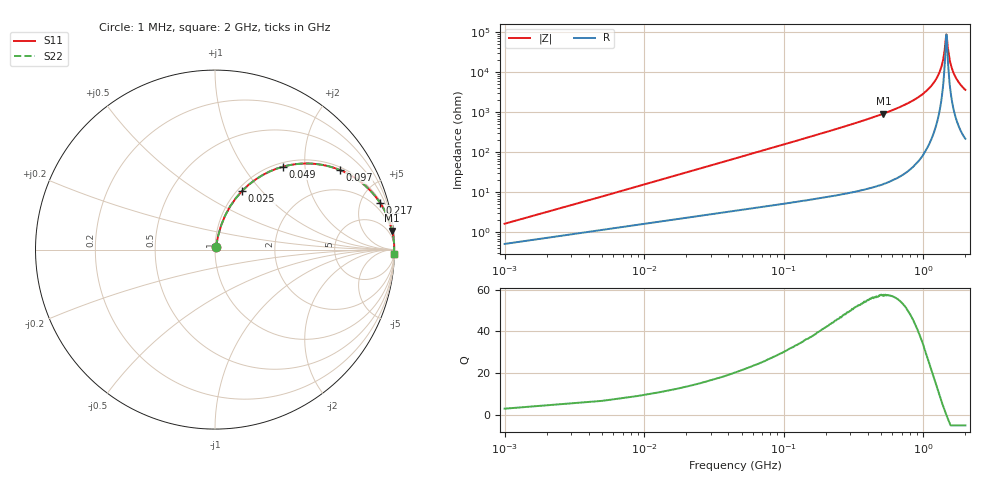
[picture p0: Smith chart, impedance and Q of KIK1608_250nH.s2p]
!version-2
!date-01.2022
!Series
# MHz S RI R 50
!Freq ReS11 ImS11 ReS21 ImS21 ReS12 ImS12 ReS22 ImS22
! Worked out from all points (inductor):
!   501 points, 1 MHz to 2 GHz, reference 50 ohm
!   read as one part in series: L = 250 nH near 9 MHz
!   highest Q = 57.5 at 517 MHz (marker M1), where L = 285 nH
!   self-resonance near 1.46 GHz
!   S11 on the Smith chart (normalised r, x): 1 MHz: 1.01, +0.03; 25 MHz: 1.05, +0.79; 49 MHz: 1.07, +1.54; 97 MHz: 1.10, +3.06; 217 MHz: 1.16, +6.97; 2 GHz: 5, -73
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1  0.00539 0.0155  0.9946 -0.0155  0.9946 -0.0155  0.00539 0.0155
13  0.0562 0.1892  0.9438 -0.1892  0.9438 -0.1892  0.0562 0.1892
25  0.1499 0.3255  0.8501 -0.3255  0.8501 -0.3255  0.1499 0.3255
49  0.3786 0.4621  0.6214 -0.4621  0.6214 -0.4621  0.3786 0.4621
97  0.695 0.4439  0.305 -0.4439  0.305 -0.4439  0.695 0.4439
145  0.8344 0.3582  0.1656 -0.3582  0.1656 -0.3582  0.8344 0.3582
217  0.9189 0.2618  0.0811 -0.2618  0.0811 -0.2618  0.9189 0.2618
337  0.9659 0.1722  0.0341 -0.1722  0.0341 -0.1722  0.9659 0.1722
517  0.9867 0.1062  0.0133 -0.1062  0.0133 -0.1062  0.9867 0.1062
669  0.993 0.0747  0.00699 -0.0747  0.00699 -0.0747  0.993 0.0747
1003  0.9979 0.0335  0.00214 -0.0335  0.00214 -0.0335  0.9979 0.0335
1210  0.9987 0.0165  0.00129 -0.0165  0.00129 -0.0165  0.9987 0.0165
1337  0.9989 0.00774  0.00112 -0.00774  0.00112 -0.00774  0.9989 0.00774
1410  0.9989 0.0032  0.00111 -0.0032  0.00111 -0.0032  0.9989 0.0032
1460  0.9989 6.81e-05  0.00113 -6.81e-05  0.00113 -6.81e-05  0.9989 6.81e-05
1470  0.9989 -0.000403  0.00114 0.000403  0.00114 0.000403  0.9989 -0.000403
1500  0.9988 -0.00227  0.00117 0.00227  0.00117 0.00227  0.9988 -0.00227
1540  0.9988 -0.00454  0.00121 0.00454  0.00121 0.00454  0.9988 -0.00454
1600  0.9987 -0.00784  0.0013 0.00784  0.0013 0.00784  0.9987 -0.00784
1670  0.9986 -0.0115  0.00143 0.0115  0.00143 0.0115  0.9986 -0.0115
1820  0.9982 -0.0191  0.00181 0.0191  0.00181 0.0191  0.9982 -0.0191
2000  0.9976 -0.0273  0.00239 0.0273  0.00239 0.0273  0.9976 -0.0273
